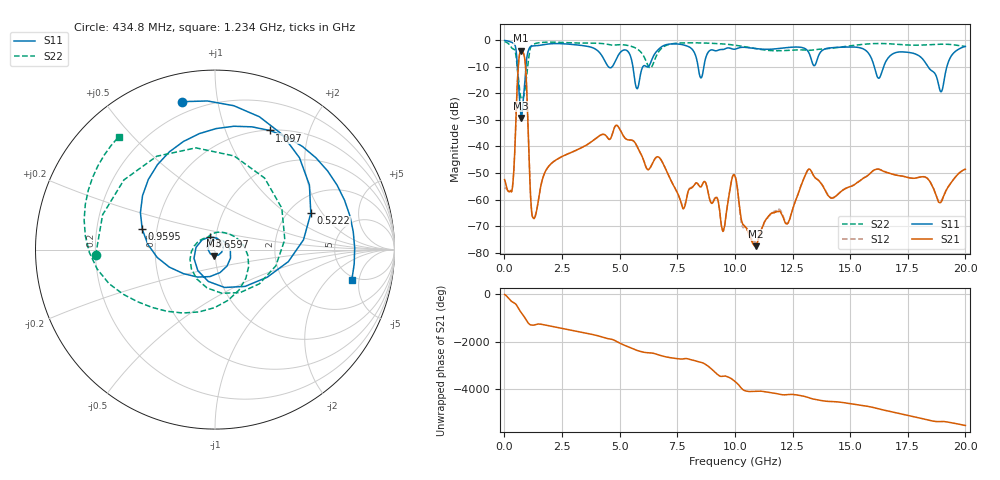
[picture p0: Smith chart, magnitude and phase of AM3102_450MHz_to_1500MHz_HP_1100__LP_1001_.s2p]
!Agilent Technologies,E8364B,MY43040894,A.07.50.67
!Agilent E8364B: A.07.50.67
!Date: Thursday, January 11, 2018 06:34:18
!Correction: S11(Full 2 Port(1,2))
!S21(Full 2 Port(1,2))
!S12(Full 2 Port(1,2))
!S22(Full 2 Port(1,2))
!S2P File: Measurements: S11, S21, S12, S22:
# Hz S  dB  R 50
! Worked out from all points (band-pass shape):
!   1601 points, 10 MHz to 20 GHz, reference 50 ohm
!   highest |S21| = -3.96 dB at 734.6 MHz (marker M1); lowest = -77.6 dB at 10.9 GHz (marker M2)
!   |S21| within 3 dB of the highest: 632.3 MHz to 882.8 MHz (250.4 MHz wide, 33.1 % of centre)
!   lowest |S11| = -29.2 dB at 734.6 MHz (marker M3), VSWR 1.07, Z = 49.4 - j3.38 ohm
!   |S11| at or under -10 dB: 5.576 GHz to 6.004 GHz (427.8 MHz wide, 7.39 % of centre); 16.05 GHz to 16.45 GHz (401.4 MHz wide, 2.47 % of centre); 18.38 GHz to 19.2 GHz (816.8 MHz wide, 4.35 % of centre)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
!   |S22| runs from -22.2 to -0.5 dB; largest |S21 - S12| = 0.00081
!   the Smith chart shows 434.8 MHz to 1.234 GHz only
!   S11 on the Smith chart (normalised r, x): 434.8 MHz: 0.14, +0.79; 522.2 MHz: 2.61, +1.56; 659.7 MHz: 0.93, +0.13; 959.5 MHz: 0.41, +0.11; 1.097 GHz: 0.51, +1.44; 1.234 GHz: 4.63, -3.97
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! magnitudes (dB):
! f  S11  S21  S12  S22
! 10 MHz  -0.1  -52.5  -55.5  -0.5
! 284.9 MHz  -0.7  -56.8  -56.8  -2.5
! 434.8 MHz  -1.5  -44.9  -45.0  -3.5
! 522.2 MHz  -4.9  -24.5  -24.4  -7.2
! 659.7 MHz  -22.3  -5.2  -5.2  -18.6
! 734.6 MHz  -29.2  -4.0  -4.0  -22.0
! 959.5 MHz  -7.5  -16.4  -16.5  -13.6
! 1.097 GHz  -2.7  -50.7  -50.5  -4.1
! 1.234 GHz  -2.1  -66.8  -66.8  -1.7
! 1.897 GHz  -1.4  -47.8  -47.7  -0.7
! 3.346 GHz  -2.0  -40.5  -40.4  -1.1
! 5.32 GHz  -3.9  -37.4  -37.4  -1.9
! 5.757 GHz  -18.2  -40.0  -40.0  -3.2
! 6.682 GHz  -3.5  -44.0  -44.0  -4.5
! 8.531 GHz  -14.2  -55.2  -55.2  -1.0
! 9.48 GHz  -3.5  -71.9  -72.1  -1.4
! 10.01 GHz  -3.4  -51.2  -51.0  -1.9
! 10.9 GHz  -3.2  -77.6  -76.3  -3.2
! 13.34 GHz  -8.0  -49.7  -49.8  -3.7
! 16.68 GHz  -6.4  -50.0  -50.0  -1.3
! 18.94 GHz  -19.4  -61.0  -60.6  -1.5
! 20 GHz  -2.3  -48.6  -48.5  -2.3
